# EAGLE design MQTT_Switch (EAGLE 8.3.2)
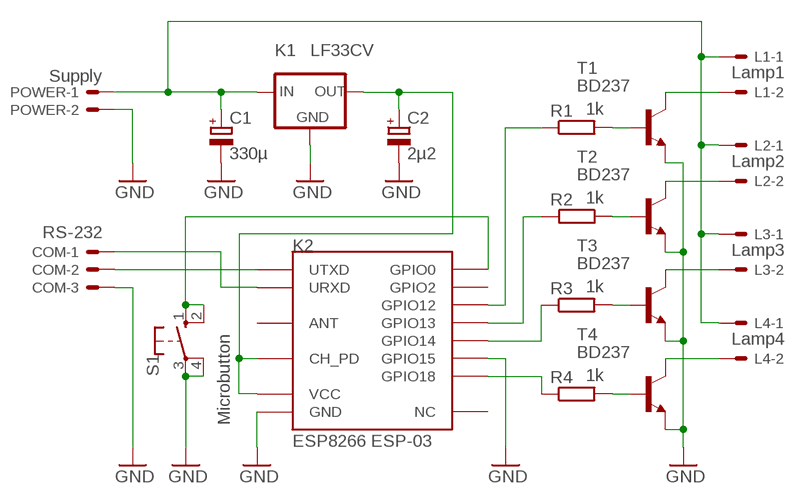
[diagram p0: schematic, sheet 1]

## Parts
C1  330µ  CPOL-EUE3.5-8  [E3,5-8]
C2  2µ2  CPOL-EUE2-5  [E2-5]
COM  RS-232  22-27-2031-03  [6410-03]
K1  LF33CV  LFXXCVS  [TO220S]
K2  ESP8266 ESP-03  ESP-03  [ESP-03]
L1  Lamp1  22-27-2021-02  [6410-02]
L2  Lamp2  22-27-2021-02  [6410-02]
L3  Lamp3  22-27-2021-02  [6410-02]
L4  Lamp4  22-27-2021-02  [6410-02]
POWER  Supply  22-27-2021-02  [6410-02]
R1  1k  R-EU_0207/10  [0207/10]
R2  1k  R-EU_0207/10  [0207/10]
R3  1k  R-EU_0207/10  [0207/10]
R4  1k  R-EU_0207/10  [0207/10]
S1  Microbutton  10-XX  [B3F-10XX]
T1  BD237  -NPN-TO126V  [TO126V]
T2  BD237  -NPN-TO126V  [TO126V]
T3  BD237  -NPN-TO126V  [TO126V]
T4  BD237  -NPN-TO126V  [TO126V]

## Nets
GND: C1.- C2.- COM.3 K1.2(GND) K2.GND K2.GPIO15 POWER.2 S1.3(P) S1.4(P1) T1.1(E) T2.1(E) T3.1(E) T4.1(E)
N$1: COM.1 K2.URXD
N$2: C1.+ K1.1(IN) L1.1 L2.1 L3.1 L4.1 POWER.1
N$3: R1.2 T1.3(B)
N$4: K2.GPIO0 S1.1(S) S1.2(S1)
N$5: R2.1 T2.3(B)
N$6: COM.2 K2.UTXD
N$7: R3.2 T3.3(B)
N$8: R4.2 T4.3(B)
N$9: K2.GPIO18 R4.1
N$10: K2.GPIO14 R3.1
N$11: C2.+ K1.3(OUT) K2.CH_PD K2.VCC
N$12: K2.GPIO13 R2.2
N$13: K2.GPIO12 R1.1
N$14: L1.2 T1.2(C)
N$15: L2.2 T2.2(C)
N$16: L3.2 T3.2(C)
N$17: L4.2 T4.2(C)
Unconnected: K2.ANT K2.GPIO2 K2.NC

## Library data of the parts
C1 C2 = rcl:CPOL-EU: POLARIZED CAPACITOR, European symbol
COM = con-molex:22-?-03: CONNECTOR wire to board 2.54 mm (.1 inch) pitch header; OC_FARNELL: unknown; OC_NEWARK: unknown
K1 = lf33:LFXXCV: VOLTAGE REGULATOR
K2 = esp8266modules:ESP-03: ESP8266 Wifi Module ESP-03; DIMENSIONS: 17.3 x 12.1 mm; PINS: 14; PITCH: 0.078" / 2 mm
L1-L4 POWER = con-molex:22-?-02: CONNECTOR; OC_FARNELL: unknown; OC_NEWARK: unknown
R1-R4 = rcl:R-EU_: RESISTOR, European symbol
S1 = switch-omron:10-XX: OMRON SWITCH
T1-T4 = transistor:*-NPN-: NPN Transistror BF959 corrected 2008.03.06

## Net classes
0 default: width 0.635 mm, clearance 0.635 mm

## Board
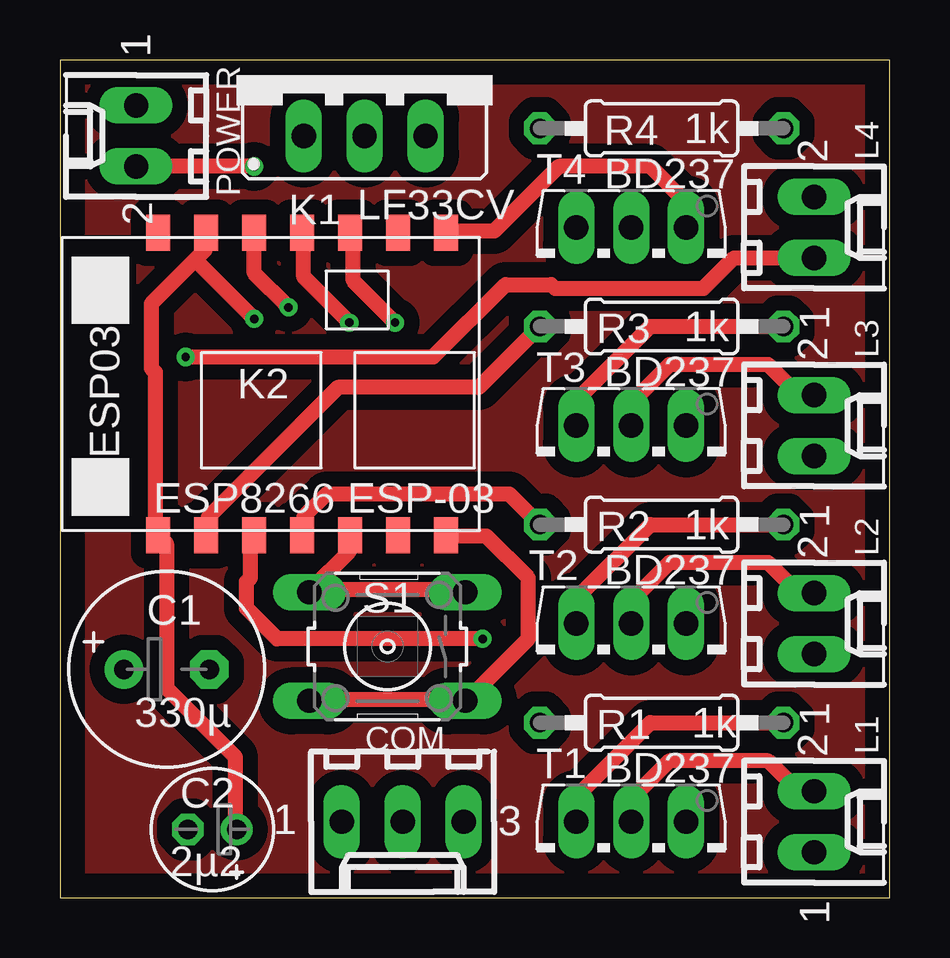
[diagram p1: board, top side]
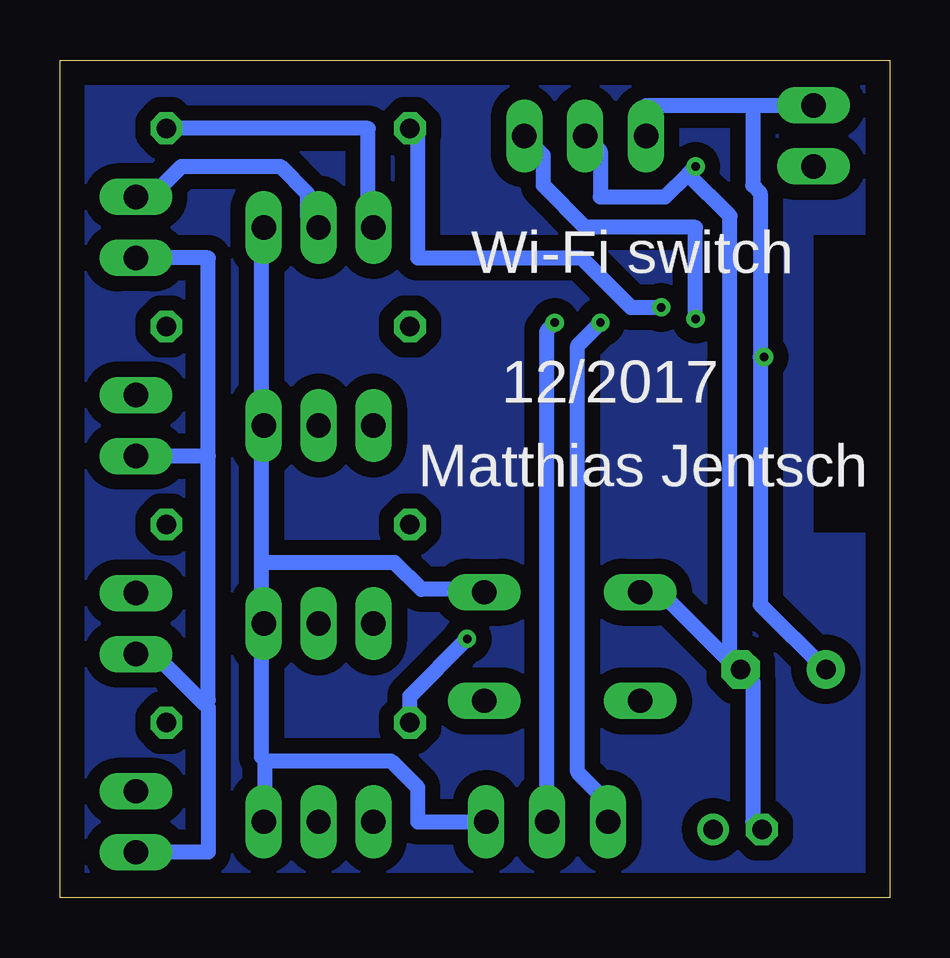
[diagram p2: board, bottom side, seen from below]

Size 34.59 x 34.91 mm. Coordinates in mm from the lower left corner, seen from the top.
Outline: 0,0 34.59,0 34.59,34.91 0,34.91 0,0
Copper layers (1*16): Top 0.035mm / dielectric 1.5mm / Bottom 0.035mm
Design rules "default": minimum track width 6mil, minimum drill 0.35mm, track to track 6mil, track to pad 6mil, pad to pad 6mil, via to via 6mil, smd to smd 6mil, copper to edge 40mil, drill to drill 6mil, minimum pad ring 10mil, minimum via ring 8mil, stop-mask expansion 4mil, vias tented up to drill 0mil, thermal gap 10mil
tRestrict: area 0,15.2 to 3.2,27.6
bRestrict: area 0,15.2 to 3.2,27.6

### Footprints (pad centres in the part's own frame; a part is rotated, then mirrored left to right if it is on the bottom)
E3,5-8 = drill 0.813 pad 1.6: + -1.778,0 | drill 0.813 pad 1.6 octagon: - 1.778,0
E2-5 = drill 0.813 pad 1.27: + -1.016,0 | drill 0.813 pad 1.27 octagon: - 1.016,0
6410-03 = drill 1.016 long: 1 2.54,0; 2 0,0; 3 -2.54,0
TO220S = drill 1.016 long: 1 -2.54,-2.54; 2 0,-2.54; 3 2.54,-2.54
ESP-03 = smd 1.5 x 1: ANT 7.4,4.8; CH_PD 7.4,2.8; GND 7.4,-7.2; GPIO0 -5.2,-7.2; GPIO2 -5.2,-5.2; GPIO12 -5.2,0.8; GPIO13 -5.2,-1.2; GPIO14 -5.2,2.8; GPIO15 -5.2,-3.2; GPIO18 7.4,0.8; NC 7.4,-5.2; URXD 7.4,-1.2; UTXD 7.4,-3.2; VCC -5.2,4.8
6410-02 = drill 1.016 long: 1 1.27,0; 2 -1.27,0
0207/10 = drill 0.813 octagon: 1 -5.08,0; 2 5.08,0
B3F-10XX = drill 1.016 long: 1 -3.251,2.261; 2 3.251,2.261; 3 -3.251,-2.261; 4 3.251,-2.261
TO126V = drill 1.016 long: 1 -2.286,-1.27; 2 0,-1.27; 3 2.286,-1.27

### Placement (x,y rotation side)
C1  4.45,9.53 0 top
C2  6.35,2.86 180 top
COM  14.29,3.17 180 top
K1  12.7,34.29 0 top
K2  8.89,20.32 90 top
L1  31.43,3.17 270 top
L2  31.43,11.43 270 top
L3  31.43,19.68 270 top
L4  31.43,27.94 270 top
POWER  3.17,31.75 90 top
R1  25.08,7.3 0 top
R2  25.08,15.56 180 top
R3  25.08,23.81 0 top
R4  25.08,32.07 0 top
S1  13.65,10.48 180 top
T1  23.81,1.91 180 top
T2  23.81,10.16 180 top
T3  23.81,18.41 180 top
T4  23.81,26.67 180 top

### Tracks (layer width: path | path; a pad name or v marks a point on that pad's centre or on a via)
GND  (via drill 0.35)
  Top 0.635: K2.GND 16.19,27.78 18.1,27.78 20.8,30.48 24.61,30.48 26.04,29.05 26.04,27.94 T4.1 | v8.1,30.48 POWER.2 | K2.GPIO15 12.06,15.08 12.06,14.45 10.48,12.86 S1.4 10.79,12.86 16.83,12.86 S1.3
  Bottom 0.635: COM.3 19.68,3.17 19.68,4.6 20.8,5.71 26.04,5.71 | 26.04,5.71 26.04,3.17 T1.1 | 26.04,5.71 26.19,5.87 26.19,11.43 T2.1 26.19,11.59 26.19,13.97 | 26.19,13.97 26.19,19.68 T3.1 26.19,19.84 26.19,27.94 T4.1 | 8.41,30.16 9.37,29.21 12.06,29.21 12.06,31.11 K1.2 | 8.41,30.16 v8.1,30.48 | C2.- 5.4,2.86 5.71,3.17 5.71,9.05 6.19,9.53 C1.- | C1.- 6.51,9.68 9.53,12.7 10.32,12.7 S1.4 | 8.41,30.16 6.67,28.42 6.67,10.16 C1.- | 26.19,13.97 20.64,13.97 19.53,12.86 16.99,12.86 S1.3
N$1  (via drill 0.35)
  Top 0.635: v12.06,23.97 10.16,25.88 10.16,27.62 K2.URXD
  Bottom 0.635: v12.06,23.97 13.02,23.02 13.02,5.24 11.75,3.97 COM.1
N$2  (via drill 0.35)
  Top 0.635: L4.1 28.1,26.67 26.83,25.4 20.64,25.4 20.48,25.56 18.57,25.56 15.56,22.54 v5.24,22.54
  Bottom 0.635: L1.1 28.42,1.91 28.42,7.94 28.57,8.1 | 28.57,8.1 30.64,10.16 L2.1 | 28.42,18.41 L3.1 | 28.42,18.41 28.42,8.26 28.57,8.1 | L4.1 28.42,26.67 28.42,18.41 | 5.71,33.02 10.16,33.02 K1.1 | 5.71,33.02 POWER.1 | 5.4,22.54 5.4,29.37 5.71,29.69 5.71,33.02 | 5.4,22.54 5.4,12.22 2.7,9.53 C1.+ | v5.24,22.54 5.4,22.54
N$3
  Top 0.635: R1.2 24.61,7.3 21.59,4.29 21.59,3.17 T1.3
N$4
  Top 0.635: K2.GPIO0 16.19,15.08 17.78,15.08 19.53,13.34 19.53,10.79 16.99,8.26 S1.1 16.67,8.26 10.48,8.26 S1.2
N$5
  Top 0.635: R2.1 24.61,15.56 21.59,12.54 21.59,11.43 T2.3
N$6  (via drill 0.35)
  Top 0.635: v13.97,23.97 12.22,25.72 12.22,27.62 K2.UTXD
  Bottom 0.635: v13.97,23.97 14.29,23.65 COM.2
N$7
  Top 0.635: R3.2 24.61,23.81 21.59,20.8 21.59,19.68 T3.3
N$8
  Bottom 0.635: R4.2 21.75,32.07 21.75,28.1 21.59,27.94 T4.3
N$9  (via drill 0.35)
  Top 0.635: v9.53,24.61 8.1,26.04 8.1,27.62 K2.GPIO18
  Bottom 0.635: v9.53,24.61 10.79,24.61 12.86,26.67 19.68,26.67 19.68,31.75 R4.1
N$10
  Top 0.635: R3.1 17.46,21.27 11.59,21.27 6.19,15.88 6.19,15.24 K2.GPIO14
N$11  (via drill 0.35)
  Top 0.635: 5.64,26.59 6.03,26.99 6.03,27.62 K2.CH_PD | 5.64,26.59 3.81,24.77 3.81,22.07 3.97,21.91 3.97,15.24 K2.VCC 4.29,14.92 4.45,14.76 4.45,8.73 7.3,5.87 7.3,2.86 C2.+ | 5.64,26.59 v8.1,24.13
  Bottom 0.635: K1.3 14.45,30.96 14.45,29.69 12.7,27.94 8.1,27.94 v8.1,24.13
N$12
  Top 0.635: R2.2 18.73,16.83 11.11,16.83 10.16,15.88 10.16,15.24 K2.GPIO13
N$13  (via drill 0.35)
  Top 0.635: v17.62,10.79 9.05,10.79 7.78,12.06 7.78,13.18 7.94,13.34 7.94,15.08 K2.GPIO12
  Bottom 0.635: v17.62,10.79 20,8.41 R1.1
N$14
  Top 0.635: T1.2 23.81,4.13 25.4,5.71 29.53,5.71 30.8,4.45 L1.2
N$15
  Top 0.635: T2.2 23.81,12.38 25.4,13.97 29.53,13.97 30.8,12.7 L2.2
N$16
  Top 0.635: T3.2 23.81,20.64 25.4,22.23 29.53,22.23 30.8,20.95 L3.2
N$17
  Bottom 0.635: T4.2 24.29,28.42 24.29,29.37 25.4,30.48 29.53,30.48 30.8,29.21 L4.2
N$18
  pour Top: -0.32,35.24 34.92,35.24 34.92,-0.32 -0.32,-0.32
N$19
  pour Bottom: -0.32,35.24 34.92,35.24 34.92,-0.32 -0.32,-0.32

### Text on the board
bNames: Wi-Fi switch | 12/2017 | Matthias Jentsch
